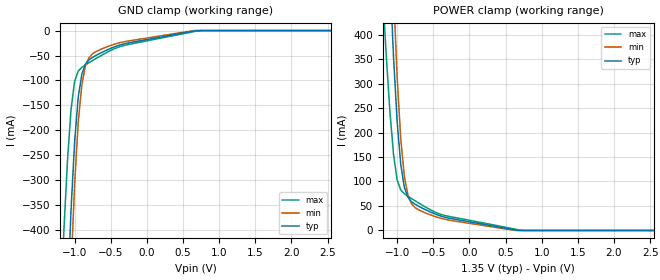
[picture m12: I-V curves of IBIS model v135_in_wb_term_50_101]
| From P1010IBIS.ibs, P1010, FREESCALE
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[Model]  v135_in_wb_term_50_101
|   Model v135_in_wb_term_50_101
| This model has derived from v135_wb_term_50_101
| Only applicable curves and parameters are copied
Model_type Input
Polarity   Non-Inverting
Enable   Active-High
Vinl =   0.5150V
Vinh =   0.9350V
C_comp   1.8439pF   1.6200pF   2.1421pF
[Receiver Thresholds]
Vth   =  0.675V
Vinh_ac  =  0.160V
Vinh_dc  =  0.090V
Vinl_ac  = -0.160V
Vinl_dc  = -0.090V
[Temperature Range]   65.0000   0.1050k   -40.0000
[Voltage Range]   1.3500V   1.2830V   1.4500V
[GND_clamp]
|Voltage   I(typ)   I(min)   I(max)
-1.45V    -2.412A    -2.862A    -1.562A
-1.15V    -758.4mA   -954.6mA   -405.7mA
-1.1V     -543mA     -701mA     -263.9mA
-1.05V    -361.5mA   -482.7mA   -159mA
-1V       -223.1mA   -308.1mA   -101.9mA
-950mV    -133.5mA   -183.8mA   -81.16mA
-900mV    -87.15mA   -108.5mA   -73.67mA
-850mV    -67.22mA   -70.66mA   -68.78mA
-750mV    -53.47mA   -46.2mA    -59.9mA
-350mV    -27.96mA   -23.49mA   -31.18mA
700mV     0A         0A         -601.8uA
2.9V      0A         0A         0A
[POWER_clamp]
|Voltage   I(typ)   I(min)   I(max)
-1.45V    2.22A      2.829A     1.239A
-1.2V     942.9mA    1.233A     485.9mA
-1.15V    723mA      956.1mA    356.7mA
-1.1V     524.6mA    705.6mA    243.5mA
-1.05V    355.1mA    488.7mA    155.7mA
-1V       223.1mA    313.9mA    103.5mA
-950mV    135.2mA    188mA      82.72mA
-900mV    88.27mA    110.8mA    74.88mA
-850mV    67.68mA    71.73mA    69.73mA
-750mV    53.41mA    46.49mA    60.4mA
750mV     0A         0A         0A
2.9V      0A         0A         0A
